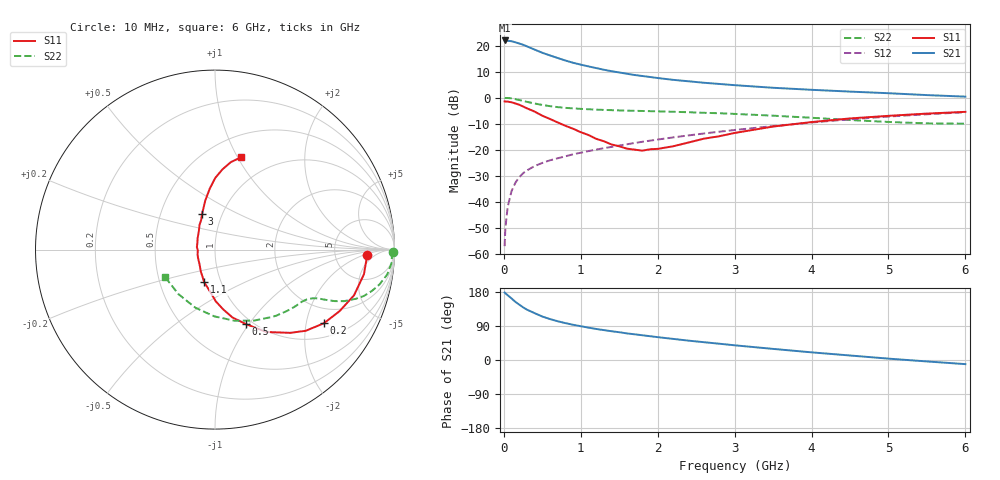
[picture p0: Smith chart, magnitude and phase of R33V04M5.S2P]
! SIEMENS Small Signal Semiconductors
! BFR181
! Si NPN RF Bipolar Junction Transistor in SOT23
! VCE = 3 V  IC = 4.5 mA
! Common Emitter S-Parameters:  May  1996
# GHz  S  MA  R  50
!  f  S11  S21  S12  S22
! GHz  MAG  ANG  MAG  ANG  MAG  ANG  MAG  ANG
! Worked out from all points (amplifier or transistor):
!   36 points, 10 MHz to 6 GHz, reference 50 ohm
!   highest |S21| = 22.0 dB at 10 MHz (marker M1)
!   |S21| within 3 dB of that: start of sweep to 359.2 MHz
!   unconditionally stable (mu >= 1): 1.173 GHz to 3.006 GHz
!   at 250 MHz: K = 0.39, MSG = 24.7 dB, |S12| = -29.0 dB
!   at 1.4 GHz: K = 1.04, MAG = 13.3 dB, |S12| = -18.9 dB
!   at 6 GHz: K = 0.86, MSG = 3.0 dB, |S12| = -5.6 dB
!   S11 on the Smith chart (normalised r, x): 10 MHz: 12, -2; 200 MHz: 1.43, -2.54; 500 MHz: 0.93, -0.97; 1.1 GHz: 0.83, -0.32; 3 GHz: 0.80, +0.33; 6 GHz: 0.72, +1.03
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0.01  0.8491 -2.0  12.59 178.1  0.0014 89.5  0.9919 -0.8
0.02  0.8456 -3.7  12.54 176.0  0.0031 95.3  0.9863 -1.7
0.05  0.8412 -9.4  12.4 170.9  0.008 81.7  0.9868 -4.3
0.1  0.8155 -18.2  12.18 162.5  0.016 82.7  0.9698 -8.2
0.15  0.7742 -26.3  11.6 153.4  0.0232 76.1  0.9365 -12.0
0.2  0.7323 -34.1  11.01 146.2  0.0296 72.4  0.9035 -14.8
0.25  0.6785 -41.8  10.41 139.0  0.0353 69.7  0.8687 -17.3
0.3  0.6251 -47.9  9.703 132.9  0.04 67.4  0.8324 -19.2
0.4  0.5408 -58.1  8.411 123.6  0.0485 64.6  0.7739 -21.8
0.5  0.4506 -67.3  7.301 114.7  0.0558 62.9  0.7254 -23.3
0.6  0.3903 -75.6  6.49 108.0  0.0626 62.4  0.6874 -24.2
0.7  0.334 -82.5  5.793 102.3  0.0685 62.2  0.6588 -24.8
0.8  0.2885 -89.1  5.182 97.3  0.0747 62.1  0.638 -25.3
1.1  0.192 -108.2  3.995 85.5  0.0941 62.7  0.5996 -27.1
1.3  0.1456 -122.9  3.448 78.9  0.1071 63.3  0.5825 -28.4
1.6  0.1048 -155.0  2.882 70.2  0.1273 63.4  0.5645 -31.0
2.2  0.1164 146.0  2.204 55.7  0.1724 62.2  0.5363 -38.1
3  0.2099 110.2  1.741 38.8  0.2393 57.9  0.488 -50.5
3.5  0.2788 101.2  1.551 29.3  0.2846 54.0  0.4514 -61.2
4.5  0.3993 89.8  1.31 11.9  0.3838 43.9  0.372 -90.6
5.5  0.4947 79.8  1.122 -3.8  0.4807 31.3  0.3209 -129.5
6  0.5344 74.3  1.048 -10.9  0.5253 24.2  0.3169 -150.8
